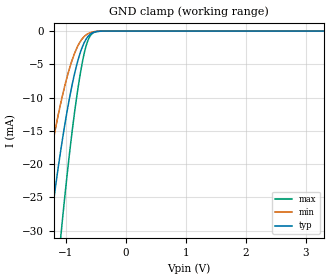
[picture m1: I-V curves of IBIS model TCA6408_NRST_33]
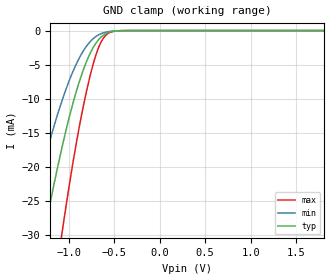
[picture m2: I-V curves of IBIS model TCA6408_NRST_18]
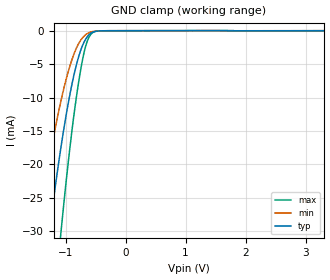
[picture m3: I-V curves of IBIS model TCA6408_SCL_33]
| TEXAS INSTRUMENTS INCORPORATED
| Standard Linear and Logic Group
| IBIS Model of TCA6408A
| LOW-VOLTAGE 8-BIT I2C AND SMBus I/O EXPANDER WITH INTERRUPT OUTPUT,
| RESET, AND CONFIGURATION REGISTERS
| This file contains package information for the following:
|  TSSOP 16-pin (PW) package as [Component] TCA6408_PW
| This device can be powered at the following Vccs:
|  5 volt Vcc
|  3.3 volt Vcc
|  2.5 volt Vcc
|  1.8 volt Vcc
| This file provides unique models under the [Model Selector] for each Vcc.
| For operation at a specific Vcc, select the appropriate model after each
| [Model Selector] keyword.
[IBIS Ver]   3.2
[Comment char]  |_char
[File Name]   tca6408a.ibs
[File Rev]   1.1 | a_die
[Date]   April 13, 2009
[Source]   Data created from TI-SPICE simulations at TI-SLL.
[Notes]   The following is an IBIS list for the TCA6408.
   Please contact sllibis@ti.com with questions and
   comments concerning SLL IBIS models.
   - FILE REV HISTORY
   - Power clamp data has been deleted as there is no
   power-clamp diode.
   - End point warning due to AC and DC mismatch.
[Disclaimer] Property of Texas Instruments Incorporated.  Unauthorized
   reproduction and/or distribution is strictly prohibited.
   This product is protected under copyright law.
   Created  2008, (C) Copyright  2008, Texas Instruments
   Incorporated, All Rights Reserved
   UNLESS THERE IS A SIGNED, WRITTEN AGREEMENT TO THE
   CONTRARY, TEXAS INSTRUMENTS (TI) IS PROVIDING THE IBIS
   MODELS  AND WITHOUT ANY WARRANTY, EXPRESSED OR
   IMPLIED.  TI assumes no liability for:
   1) the accuracy of the IBIS models provided to your
   company;
   2) the proper functioning of these IBIS Models in your
   design or for any resulting applications; or
   3) infringement of patents, copyrights or intellectual
   property rights resulting from your use of these IBIS
   models.
   TI provides IBIS Models as a service to our customers.
   You and your company shall not distribute, sell or give
   these models to anyone else without prior written
   permission from TI.
   TI reserves the right to make changes to our products or
   to discontinue any semiconductor product or service
   without notice, and advises our customers to obtain the
   latest version of relevant information to verify, before
   placing orders, that the information being relied on is
   current.
   Please be aware that your receipt and use of the IBIS
   information provided shall serve as acceptance of these
   terms and conditions.  If you do not accept these terms,
   you should return or destroy the IBIS models and any
   other accompanying information immediately.
| Component TCA6408_PW 16-PIN TSSOP
[Component]   TCA6408_PW
[Manufacturer]   Texas Instruments, Inc.
[Package]
|   typ   min   max
R_pkg   4.500e-02   3.800e-02   5.100e-02
L_pkg   2.593e-09   2.447e-09   3.080e-09
C_pkg   2.810e-13   2.430e-13   3.770e-13
[Pin]   signal_name   model_name   R_pin   L_pin   C_pin
1   VCCI   POWER   4.000e-02   3.080e-09   3.770e-13
2   ADDR   TCA6408_ADDR   3.800e-02   2.458e-09   2.810e-13
3   NRESET   TCA6408_NRST   5.100e-02   2.512e-09   2.550e-13
4   P0   TCA6408_P   5.100e-02   2.447e-09   2.430e-13
5   P1   TCA6408_P   5.100e-02   2.447e-09   2.430e-13
6   P2   TCA6408_P   5.100e-02   2.512e-09   2.550e-13
7   P3   TCA6408_P   3.800e-02   2.458e-09   2.810e-13
8   GND   GND   4.000e-02   3.080e-09   3.770e-13
9   P4   TCA6408_P   3.900e-02   2.832e-09   3.160e-13
10   P5   TCA6408_P   3.800e-02   2.460e-09   2.790e-13
11   P6   TCA6408_P   5.100e-02   2.512e-09   2.550e-13
12   P7   TCA6408_P   5.100e-02   2.447e-09   2.430e-13
13   NINT   TCA6408_NINT   5.100e-02   2.447e-09   2.430e-13
14   SCL   TCA6408_SCL   5.100e-02   2.512e-09   2.550e-13
15   SDA   TCA6408_SDA   3.800e-02   2.459e-09   2.790e-13
16   VCCP   POWER   3.900e-02   2.832e-09   3.160e-13
| Model TCA6408_NRST
[Model Selector]   TCA6408_NRST
TCA6408_NRST_50   5 volt Vcc
TCA6408_NRST_33   3.3 volt Vcc
TCA6408_NRST_25   2.5 volt Vcc
TCA6408_NRST_18   1.8 volt Vcc
| Model TCA6408_SCL
[Model Selector]   TCA6408_SCL
TCA6408_SCL_50   5 volt Vcc
TCA6408_SCL_33   3.3 volt Vcc
TCA6408_SCL_25   2.5 volt Vcc
TCA6408_SCL_18   1.8 volt Vcc
| Model TCA6408_ADDR
[Model Selector]   TCA6408_ADDR
TCA6408_ADDR_50   5 volt Vcc
TCA6408_ADDR_33   3.3 volt Vcc
TCA6408_ADDR_25   2.5 volt Vcc
TCA6408_ADDR_18   1.8 volt Vcc
| Model TCA6408_P
[Model Selector]   TCA6408_P
TCA6408_P_50   5 volt Vcc
TCA6408_P_33   3.3 volt Vcc
TCA6408_P_25   2.5 volt Vcc
TCA6408_P_18   1.8 volt Vcc
| Model TCA6408_SDA
[Model Selector]   TCA6408_SDA
TCA6408_SDA_50   5 volt Vcc
TCA6408_SDA_33   3.3 volt Vcc
TCA6408_SDA_25   2.5 volt Vcc
TCA6408_SDA_18   1.8 volt Vcc
| Model TCA6408_NINT
[Model Selector]   TCA6408_NINT
TCA6408_NINT_50   5 volt Vcc
TCA6408_NINT_33   3.3 volt Vcc
TCA6408_NINT_25   2.5 volt Vcc
TCA6408_NINT_18   1.8 volt Vcc
| Models and submodels in the file (24): TCA6408_NRST_50 (Input), TCA6408_NRST_33 (Input), TCA6408_NRST_25 (Input), TCA6408_NRST_18 (Input), TCA6408_SCL_50 (Input), TCA6408_SCL_33 (Input), TCA6408_SCL_25 (Input), TCA6408_SCL_18 (Input), TCA6408_ADDR_50 (Input), TCA6408_ADDR_33 (Input), TCA6408_ADDR_25 (Input), TCA6408_ADDR_18 (Input), TCA6408_P_50 (I/O), TCA6408_P_33 (I/O), TCA6408_P_25 (I/O), TCA6408_P_18 (I/O), TCA6408_SDA_50 (I/O_open_drain), TCA6408_SDA_33 (I/O_open_drain), TCA6408_SDA_25 (I/O_open_drain), TCA6408_SDA_18 (I/O_open_drain), TCA6408_NINT_50 (Open_drain), TCA6408_NINT_33 (Open_drain), TCA6408_NINT_25 (Open_drain), TCA6408_NINT_18 (Open_drain)
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[Model]   TCA6408_NRST_33
Model_type  Input
Vinl=0.9
Vinh=2.52
| variable   typ   min   max
C_comp   2.22pF   1.76pF   2.42pF
[Temperature Range]   40   100   -40
| Ambient temperature   25   85   -40
[Voltage range]   3.3   3   3.6
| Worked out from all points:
|   GND clamp passes 1 mA (typ) near -0.65 V on its own axis
[GND Clamp]
| TCA6408_NRST_33
|   Voltage   I(typ)   I(min)   I(max)
-3.3V     -229.8mA   -173.1mA   -314.8mA
-1.49V    -47mA      -31.57mA   -73.96mA
-1.455V   -44.17mA   -29.5mA    -69.9mA
-1.285V   -31.19mA   -20.13mA   -51.01mA
-1.255V   -29.05mA   -18.6mA    -47.84mA
-1.08V    -17.66mA   -10.65mA   -30.52mA
-945mV    -10.37mA   -5.81mA    -18.9mA
-810mV    -4.799mA   -2.428mA   -9.366mA
-700mV    -1.861mA   -882.4uA   -3.61mA
-615mV    -655uA     -320.4uA   -1.07mA
-410mV    -13.36uA   -10.66uA   -11.01uA
3.3V      289.3pA    1.025nA    57.78pA
[Model]   TCA6408_NRST_18
Model_type  Input
Vinl=0.495
Vinh=1.365
| variable   typ   min   max
C_comp   2.21pF   1.67pF   2.46pF
[Temperature Range]   40   100   -40
| Ambient temperature   25   85   -40
[Voltage range]   1.8   1.65   1.95
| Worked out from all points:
|   GND clamp passes 1 mA (typ) near -0.65 V on its own axis
[GND Clamp]
| TCA6408_NRST_18
|   Voltage   I(typ)   I(min)   I(max)
-1.8V     -74.02mA   -51.67mA   -111.7mA
-1.45V    -43.77mA   -29.21mA   -69.33mA
-1.27V    -30.12mA   -19.36mA   -49.42mA
-1.25V    -28.7mA    -18.35mA   -47.31mA
-1.07V    -17.07mA   -10.25mA   -29.6mA
-960mV    -11.11mA   -6.281mA   -20.1mA
-855mV    -6.438mA   -3.375mA   -12.27mA
-765mV    -3.406mA   -1.667mA   -6.757mA
-680mV    -1.498mA   -708.4uA   -2.836mA
-590mV    -450.5uA   -228.8uA   -677.8uA
-475mV    -54.97uA   -37.86uA   -56.06uA
1.8V      147.6pA    546pA      30.99pA
[Model]   TCA6408_SCL_33
Model_type  Input
Vinl=0.9
Vinh=2.52
| variable   typ   min   max
C_comp   2.17pF   1.72pF   2.37pF
[Temperature Range]   40   100   -40
| Ambient temperature   25   85   -40
[Voltage range]   3.3   3   3.6
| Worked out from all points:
|   GND clamp passes 1 mA (typ) near -0.65 V on its own axis
[GND Clamp]
| TCA6408_SCL_33
|   Voltage   I(typ)   I(min)   I(max)
-3.3V     -229.8mA   -173.1mA   -314.8mA
-1.49V    -47.01mA   -31.58mA   -73.96mA
-1.455V   -44.17mA   -29.5mA    -69.91mA
-1.285V   -31.2mA    -20.13mA   -51.01mA
-1.255V   -29.06mA   -18.61mA   -47.84mA
-1.08V    -17.66mA   -10.65mA   -30.52mA
-945mV    -10.38mA   -5.815mA   -18.91mA
-810mV    -4.804mA   -2.432mA   -9.37mA
-700mV    -1.866mA   -886.6uA   -3.615mA
-615mV    -659.7uA   -324.3uA   -1.075mA
-400mV    -14.1uA    -11.42uA   -12.78uA
3.3V      289.3pA    2.092uA    -3.305uA
